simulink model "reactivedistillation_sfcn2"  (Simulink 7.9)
settings: Solver=ode15s  StartTime=t0  StopTime=tfin  MinStep=1e-9  RelTol=1e-9
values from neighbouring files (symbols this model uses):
  B = block.InputPort(6).Data    [Distillation_sfcn2.m]    (also in main_script.m = 209.95; reactive_distDAE.m = 244.9)
  Con_set = 25    [main_script.m]
  D = block.InputPort(3).Data    [Distillation_sfcn2.m]    (also in main_script.m = 140.05; reactive_distDAE.m = 105)
  F0 = block.InputPort(1).Data    [Distillation_sfcn2.m]    (also in main_script.m = sum(F); reactive_distDAE.m = sum(F))
  Ntrays = 20    [Distillation_sfcn2.m]    (also in main_script.m; reactive_distDAE.m)
  Reb_set = 25    [main_script.m]
  Ref = block.InputPort(5).Data    [Distillation_sfcn2.m]    (also in main_script.m = 3; reactive_distDAE.m = 315)
  Vb = block.InputPort(4).Data    [Distillation_sfcn2.m]    (also in main_script.m = 430; reactive_distDAE.m = 430)
  x_in = block.InputPort(2).Data    [Distillation_sfcn2.m]    (also in main_script.m = F/F0; reactive_distDAE.m = F/F0)
  x_new = F_new/F0    [main_script.m]
libraries: simulink x2

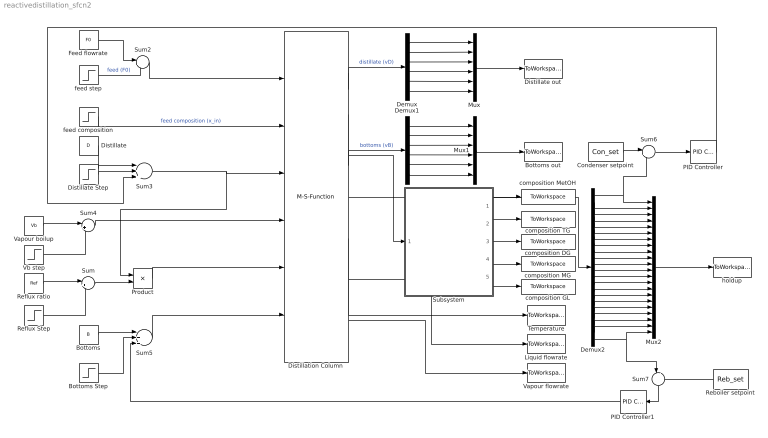
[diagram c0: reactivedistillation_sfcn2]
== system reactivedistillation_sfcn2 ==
  Bottoms : Constant  Value=B
  Bottoms Step : Step  After=0  SampleTime=0
  Bottoms out : ToWorkspace  VariableName=Bottoms  SampleTime=-1  SaveFormat=Structure With Time
  Condenser setpoint : Constant  Value=Con_set
  Demux : Demux  Outputs=6
  Demux1 : Demux  Outputs=6
  Demux2 : Demux  Outputs=22
  Distillate : Constant  Value=D
  Distillate Step : Step  After=0.1*D*0  SampleTime=0
  Distillate out : ToWorkspace  VariableName=Distillate  SampleTime=-1  SaveFormat=Structure With Time
  Distillation Column : M-S-Function  FunctionName=Distillation_sfcn2
  Feed flowrate : Constant  Value=F0
  Liquid flowrate : ToWorkspace  VariableName=L_flow  SampleTime=-1  SaveFormat=Structure With Time
  Mux : Mux  Inputs=6
  Mux1 : Mux  Inputs=6
  Mux2 : Mux  Inputs=22
  PID Controller : simulink/Continuous/PID Controller  Controller=P  TimeDomain=Continuous-time  SampleTime=1  IntegratorMethod=Forward Euler  FilterMethod=Forward Euler  Form=Parallel  P=-10  I=1  D=0  N=100  InitialConditionSource=internal  InitialConditionForIntegrator=0  InitialConditionForFilter=0  ExternalReset=none  LimitOutput=off  UpperSaturationLimit=inf  LowerSaturationLimit=-inf  LinearizeAsGain=off  AntiWindupMode=none  Kb=1  TrackingMode=off  Kt=1  PParamMin=[]  PParamMax=[]  IParamMin=[]  IParamMax=[]  DParamMin=[]  DParamMax=[]  NParamMin=[]  NParamMax=[]  KbParamMin=[]  KbParamMax=[]  KtParamMin=[]  KtParamMax=[]  POutMin=[]  POutMax=[]  IOutMin=[]  IOutMax=[]  DOutMin=[]  DOutMax=[]  NOutMin=[]  NOutMax=[]  KbOutMin=[]  KbOutMax=[]  KtOutMin=[]  KtOutMax=[]  IntegratorOutMin=[]  IntegratorOutMax=[]  FilterOutMin=[]  FilterOutMax=[]  SumOutMin=[]  SumOutMax=[]  SumI1OutMin=[]  SumI1OutMax=[]  SumI2OutMin=[]  SumI2OutMax=[]  SumI3OutMin=[]  SumI3OutMax=[]  SumDOutMin=[]  SumDOutMax=[]  SaturationOutMin=[]  SaturationOutMax=[]  IntegratorContinuousStateAttributes=''  IntegratorStateMustResolveToSignalObject=off  IntegratorRTWStateStorageClass=Auto  FilterContinuousStateAttributes=''  FilterStateMustResolveToSignalObject=off  FilterRTWStateStorageClass=Auto
  PID Controller1 : simulink/Continuous/PID Controller  Controller=P  TimeDomain=Continuous-time  SampleTime=1  IntegratorMethod=Forward Euler  FilterMethod=Forward Euler  Form=Parallel  P=-10  I=1  D=0  N=100  InitialConditionSource=internal  InitialConditionForIntegrator=0  InitialConditionForFilter=0  ExternalReset=none  LimitOutput=off  UpperSaturationLimit=inf  LowerSaturationLimit=-inf  LinearizeAsGain=off  AntiWindupMode=none  Kb=1  TrackingMode=off  Kt=1  PParamMin=[]  PParamMax=[]  IParamMin=[]  IParamMax=[]  DParamMin=[]  DParamMax=[]  NParamMin=[]  NParamMax=[]  KbParamMin=[]  KbParamMax=[]  KtParamMin=[]  KtParamMax=[]  POutMin=[]  POutMax=[]  IOutMin=[]  IOutMax=[]  DOutMin=[]  DOutMax=[]  NOutMin=[]  NOutMax=[]  KbOutMin=[]  KbOutMax=[]  KtOutMin=[]  KtOutMax=[]  IntegratorOutMin=[]  IntegratorOutMax=[]  FilterOutMin=[]  FilterOutMax=[]  SumOutMin=[]  SumOutMax=[]  SumI1OutMin=[]  SumI1OutMax=[]  SumI2OutMin=[]  SumI2OutMax=[]  SumI3OutMin=[]  SumI3OutMax=[]  SumDOutMin=[]  SumDOutMax=[]  SaturationOutMin=[]  SaturationOutMax=[]  IntegratorContinuousStateAttributes=''  IntegratorStateMustResolveToSignalObject=off  IntegratorRTWStateStorageClass=Auto  FilterContinuousStateAttributes=''  FilterStateMustResolveToSignalObject=off  FilterRTWStateStorageClass=Auto
  Product : Product
  Reboiler setpoint : Constant  Value=Reb_set
  Reflux Step : Step  After=0  SampleTime=0
  Reflux ratio : Constant  Value=Ref
  Subsystem : Subsystem
  Sum : Sum  Inputs=|++
  Sum2 : Sum  Inputs=|++
  Sum3 : Sum  Inputs=|+++
  Sum4 : Sum  Inputs=|++
  Sum5 : Sum  Inputs=|+++
  Sum6 : Sum  Inputs=|+-
  Sum7 : Sum  Inputs=|-+
  Temperature : ToWorkspace  VariableName=Temp  SampleTime=-1
  Vapour boilup : Constant  Value=Vb
  Vapour flowrate : ToWorkspace  VariableName=V_flow  SampleTime=-1  SaveFormat=Structure With Time
  Vb step : Step  After=Vb*0.1*0  SampleTime=0
  composition DG : ToWorkspace  VariableName=x_DG  SampleTime=-1
  composition GL : ToWorkspace  VariableName=x_GL  SampleTime=-1
  composition MG : ToWorkspace  VariableName=x_MG  SampleTime=-1
  composition MetOH : ToWorkspace  VariableName=x_MetOH  SampleTime=-1
  composition TG : ToWorkspace  VariableName=x_TG  SampleTime=-1
  feed composition : Step  Time=10  Before=x_in  After=x_new  SampleTime=0
  feed step : Step  Time=10  After=F0*0.10*0  SampleTime=0
  holdup : ToWorkspace  VariableName=H_out  SampleTime=-1  SaveFormat=Structure With Time
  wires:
  Distillation Column/1 -> Demux/1  "distillate (vD)"
  Distillation Column/2 -> Demux1/1  "bottoms (vB)"
  Distillation Column/3 -> Subsystem/1(In1)
  Demux/2 -> Mux/2
  Mux/1 -> Distillate out/1
  Demux/3 -> Mux/3
  Demux/4 -> Mux/4
  Demux/5 -> Mux/5
  Demux/6 -> Mux/6
  Demux1/1 -> Mux1/1
  Demux1/2 -> Mux1/2
  Mux1/1 -> Bottoms out/1
  Demux1/3 -> Mux1/3
  Demux1/4 -> Mux1/4
  Demux1/5 -> Mux1/5
  Demux1/6 -> Mux1/6
  Subsystem/1(Out1) -> composition MetOH/1
  Subsystem/2(Out2) -> composition TG/1
  Subsystem/3(Out3) -> composition DG/1
  Subsystem/4(Out4) -> composition MG/1
  Subsystem/5(Out5) -> composition GL/1
  Distillation Column/4 -> Demux2/1
  Demux2/1 -> Mux2/1, Sum6/2
  Demux2/2 -> Mux2/2
  Demux2/3 -> Mux2/3
  Demux2/4 -> Mux2/4
  Demux2/5 -> Mux2/5
  Demux2/6 -> Mux2/6
  Demux2/7 -> Mux2/7
  Demux2/8 -> Mux2/8
  Demux2/9 -> Mux2/9
  Demux2/10 -> Mux2/10
  Demux2/11 -> Mux2/11
  Demux2/12 -> Mux2/12
  Demux2/13 -> Mux2/13
  Demux2/14 -> Mux2/14
  Demux2/15 -> Mux2/15
  Demux2/16 -> Mux2/16
  Demux2/17 -> Mux2/17
  Demux2/18 -> Mux2/18
  Demux2/19 -> Mux2/19
  Demux2/20 -> Mux2/20
  Demux2/21 -> Mux2/21
  Demux2/22 -> Mux2/22, Sum7/1
  Mux2/1 -> holdup/1
  Feed flowrate/1 -> Sum2/1
  Distillate/1 -> Sum3/1
  Distillate Step/1 -> Sum3/2
  Sum3/1 -> Distillation Column/3, Product/1
  Vapour boilup/1 -> Sum4/1
  Demux/1 -> Mux/1
  feed step/1 -> Sum2/2  "feed (F0)"
  Sum2/1 -> Distillation Column/1
  Distillation Column/5 -> Temperature/1
  Distillation Column/6 -> Liquid flowrate/1
  Bottoms/1 -> Sum5/1
  Bottoms Step/1 -> Sum5/2
  Sum5/1 -> Distillation Column/6
  Distillation Column/7 -> Vapour flowrate/1
  Sum6/1 -> PID Controller/1
  Sum7/1 -> PID Controller1/1
  Reboiler setpoint/1 -> Sum7/2
  PID Controller1/1 -> Sum5/3
  Condenser setpoint/1 -> Sum6/1
  PID Controller/1 -> Sum3/3
  Reflux ratio/1 -> Sum/1
  Reflux Step/1 -> Sum/2
  Sum/1 -> Product/2
  Product/1 -> Distillation Column/5
  Vb step/1 -> Sum4/2
  Sum4/1 -> Distillation Column/4
  feed composition/1 -> Distillation Column/2  "feed composition (x_in)"

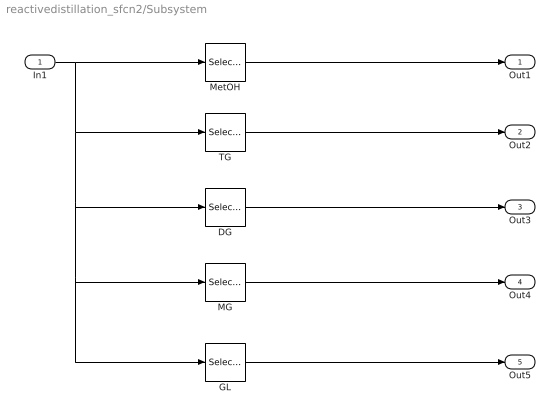
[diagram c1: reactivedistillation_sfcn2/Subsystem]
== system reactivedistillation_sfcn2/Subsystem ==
  In1 : Inport
  DG : Selector  InputPortWidth=(Ntrays+2)*5  IndexOptions=Index vector (dialog)  Indices=[45:66]  OutputSizes=1
  GL : Selector  InputPortWidth=(Ntrays+2)*5  IndexOptions=Index vector (dialog)  Indices=[89:110]  OutputSizes=1
  MG : Selector  InputPortWidth=(Ntrays+2)*5  IndexOptions=Index vector (dialog)  Indices=[67:88]  OutputSizes=1
  MetOH : Selector  InputPortWidth=(Ntrays+2)*5  IndexOptions=Index vector (dialog)  Indices=[1:22]  OutputSizes=1
  TG : Selector  InputPortWidth=(Ntrays+2)*5  IndexOptions=Index vector (dialog)  Indices=[23:44]  OutputSizes=1
  Out1 : Outport
  Out2 : Outport  Port=2
  Out3 : Outport  Port=3
  Out4 : Outport  Port=4
  Out5 : Outport  Port=5
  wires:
  In1/1 -> MetOH/1, TG/1, DG/1, MG/1, GL/1
  MetOH/1 -> Out1/1
  TG/1 -> Out2/1
  DG/1 -> Out3/1
  MG/1 -> Out4/1
  GL/1 -> Out5/1
